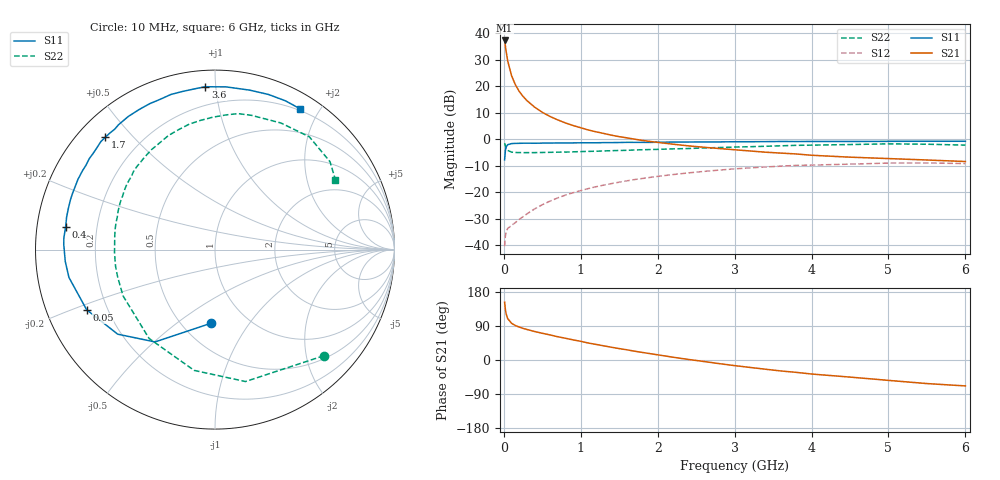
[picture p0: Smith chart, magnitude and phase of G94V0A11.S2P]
! SIEMENS Small Signal Semiconductors
! BFG235
! Si NPN RF Bipolar Junction Transistor in SOT223
! VCE = 4 V  IC = 110 mA
! Common Emitter S-Parameters:  July  1994
# GHz  S  MA  R  50
!  f  S11  S21  S12  S22
! GHz  MAG  ANG  MAG  ANG  MAG  ANG  MAG  ANG
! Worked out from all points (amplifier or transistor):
!   40 points, 10 MHz to 6 GHz, reference 50 ohm
!   highest |S21| = 37.2 dB at 10 MHz (marker M1)
!   |S21| within 3 dB of that: start of sweep to 24.37 MHz
!   unconditionally stable (mu >= 1): 460.8 MHz to 1.502 GHz
!   at 200 MHz: K = 0.78, MSG = 24.1 dB, |S12| = -30.2 dB
!   at 1.5 GHz: K = 1.00, MAG = 8.4 dB, |S12| = -16.2 dB
!   at 6 GHz: K = 0.91, MSG = 0.4 dB, |S12| = -9.2 dB
!   S11 on the Smith chart (normalised r, x): 10 MHz: 0.68, -0.68; 50 MHz: 0.12, -0.22; 400 MHz: 0.09, +0.08; 1.7 GHz: 0.08, +0.42; 3.6 GHz: 0.09, +0.94; 6 GHz: 0.18, +1.76
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0.01  0.4111 -93.2  72.57 152.6  0.0097 63.0  0.8468 -44.3
0.02  0.6134 -123.0  57.06 133.7  0.015 49.8  0.7544 -77.0
0.03  0.7183 -139.0  44.88 121.9  0.0183 41.2  0.6829 -99.8
0.05  0.7898 -154.9  29.93 109.2  0.0209 33.2  0.6163 -126.6
0.1  0.8284 -169.2  15.83 97.0  0.0238 35.6  0.5736 -153.3
0.15  0.8369 -175.5  10.63 90.9  0.027 41.4  0.5634 -164.4
0.2  0.8387 -178.8  7.953 86.9  0.031 45.2  0.5617 -170.6
0.25  0.8431 178.1  6.411 83.4  0.0349 49.5  0.5596 -174.9
0.3  0.8445 175.6  5.352 80.6  0.0392 52.1  0.5601 -178.5
0.4  0.8418 171.3  4.029 75.2  0.0488 55.3  0.5603 176.4
0.5  0.8464 167.6  3.218 70.5  0.0585 56.7  0.5639 172.1
0.6  0.8485 164.5  2.686 66.2  0.0684 57.1  0.5677 168.4
0.7  0.852 160.9  2.317 61.4  0.0787 56.7  0.5715 164.9
0.9  0.8547 155.5  1.816 53.1  0.0984 54.2  0.58 158.7
1.1  0.8592 149.1  1.492 44.7  0.118 51.1  0.5913 152.6
1.7  0.8749 134.3  1.004 23.2  0.1743 39.1  0.6286 136.3
2.2  0.8852 123.1  0.807 7.3  0.2164 28.0  0.6594 122.7
3.2  0.8995 101.6  0.602 -19.6  0.2889 4.8  0.7241 96.6
3.6  0.9091 93.4  0.549 -28.9  0.3114 -5.1  0.7527 85.4
4.5  0.9092 77.8  0.46 -45.1  0.3402 -25.0  0.7952 62.5
5.5  0.9171 64.7  0.407 -62.2  0.3583 -46.9  0.8065 37.4
6  0.9168 58.7  0.381 -68.4  0.3485 -55.0  0.7759 30.2
